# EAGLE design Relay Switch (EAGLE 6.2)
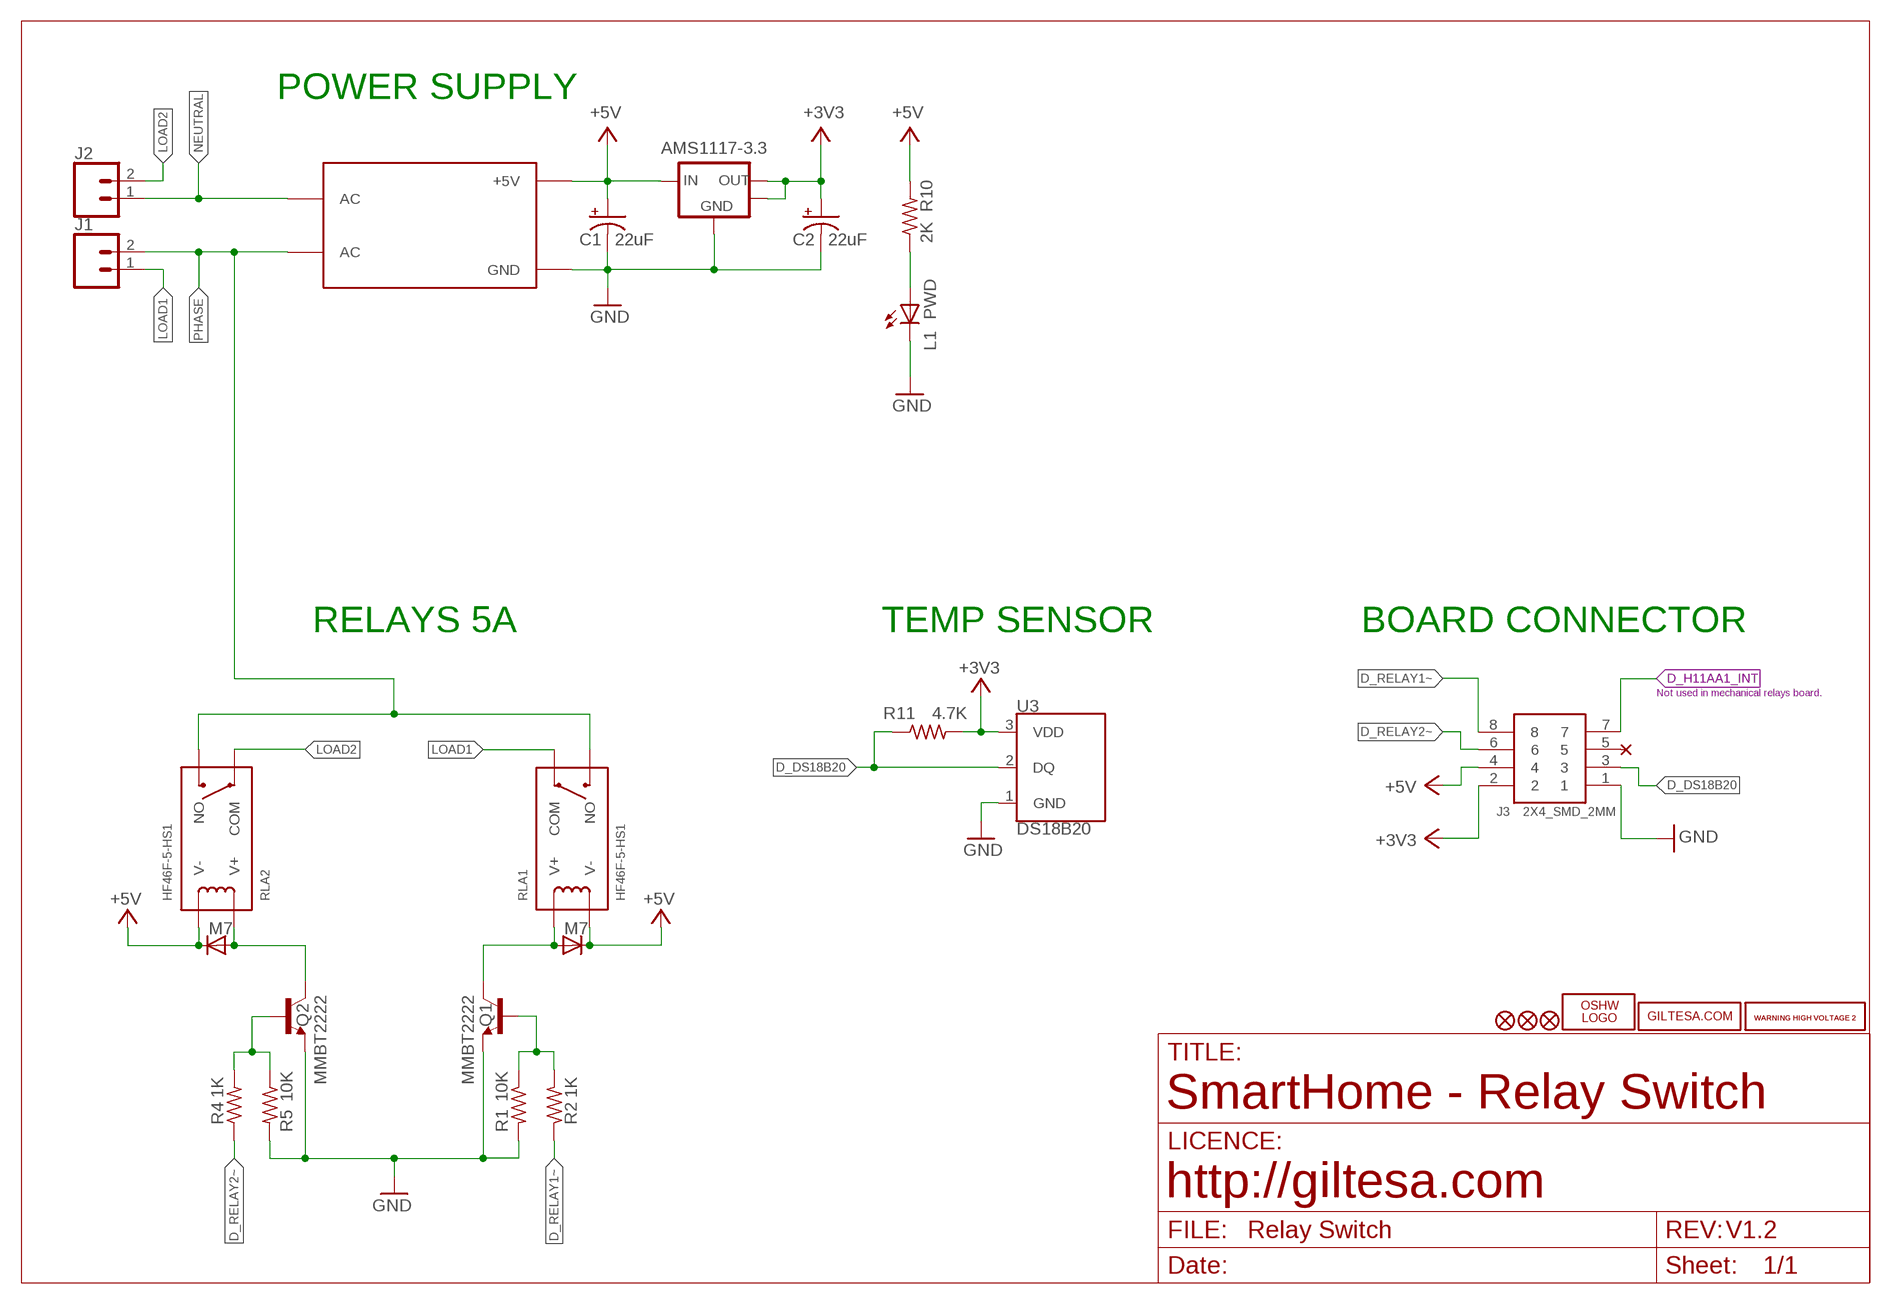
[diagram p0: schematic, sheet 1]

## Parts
AMS1117-3.3  AMS1117-3.3  AMS1117SOT89_2  [SOT89_2]
C1  22uF  CAP_POL3528  [EIA3528]
C2  22uF  CAP_POL3528  [EIA3528]
D1  M7  DIODE-SMB  [SMB]
D2  M7  DIODE-SMB  [SMB]
J1  TERMINAL_5MM_2P_90º  [TERMINAL_5MM_2P_90º]
J2  TERMINAL_5MM_2P_90º  [TERMINAL_5MM_2P_90º]
J3  2X4_SMD_2MM  2X4_SMD_2.0MM  [2X4_SMD_2.0MM]
L1  PWD  LEDCHIP-LED0805  [CHIP-LED0805]
LOGO1  OSHW_LOGO_FILLX0150-NT  [OSHW_FILLX150_NOTEXT]
Q1  MMBT2222  TRANSISTOR_NPNSOT23  [SOT23]
Q2  MMBT2222  TRANSISTOR_NPNSOT23  [SOT23]
R1  10K  R0603  [R0603]
R2  1K  R0603  [R0603]
R4  1K  R0603  [R0603]
R5  10K  R0603  [R0603]
R10  2K  R0603  [R0603]
R11  4.7K  R0603  [R0603]
RLA1  HF46F-5-HS1  RELAY_HF46F-5-HS1  [RELAY_HF46F-5-HS1]
RLA2  HF46F-5-HS1  RELAY_HF46F-5-HS1  [RELAY_HF46F-5-HS1]
U3  DS18B20  [DS18B20]
U$1  HILINK_HLK-PM01_5V  [HILINK_HLK-PM01_5V]
U$3  WARNING_HIGH_VOLTAGE_2  [WARNING_HIGH_VOLTAGE_2]
U$4  WARNING_HIGH_VOLTAGE_2  [WARNING_HIGH_VOLTAGE_2]
U$5  GILTESA.COM_MASK  [GILTESA.COM_MASK]
U$6  FIDUCIAL1X2  [FIDUCIAL-1X2]
U$7  FIDUCIAL1X2  [FIDUCIAL-1X2]
U$14  FIDUCIAL1X2  [FIDUCIAL-1X2]

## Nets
+3V3: AMS1117-3.3.2(OUT) AMS1117-3.3.4(NC) C2.A(+) J3.2 R11.2 U3.3(VDD)
+5V: AMS1117-3.3.3(IN) C1.A(+) D1.C D2.C J3.4 R10.2 RLA1.V- RLA2.V- U$1.+5V
D_DS18B20: J3.3 R11.1 U3.2(DQ)
D_H11AA1_INT: J3.7
D_RELAY1~: J3.8 R2.1
D_RELAY2~: J3.6 R4.1
GND: AMS1117-3.3.1(GND) C1.C(-) C2.C(-) J3.1 L1.C Q1.2(E) Q2.2(E) R1.2 R5.2 U3.1(GND) U$1.GND
LOAD1: J1.1 RLA1.COM
LOAD2: J2.2 RLA2.COM
N$2: Q1.1(B) R1.1 R2.2
N$3: D1.A Q1.3(C) RLA1.V+
N$8: L1.A R10.1
N$46: Q2.1(B) R4.2 R5.1
N$47: D2.A Q2.3(C) RLA2.V+
NEUTRAL: J2.1 U$1.AC@2(AC)
PHASE: J1.2 RLA1.NO RLA2.NO U$1.AC@1(AC)
Unconnected: J3.5

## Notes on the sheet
- POWER SUPPLY
- RELAYS 5A | TEMP SENSOR | BOARD CONNECTOR
- Not used in mechanical relays board.
- SmartHome - Relay Switch
- http://giltesa.com
- V1.2

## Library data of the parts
AMS1117-3.3 = ,giltesa:AMS1117
C1 C2 = SparkFun:CAP_POL: Capacitor Polarized
D1 D2 = diode:DIODE-: DIODE
J1 J2 = ,giltesa:TERMINAL_5MM_2P_90º
J3 = ,giltesa:2X4_SMD_2.0MM
L1 = led:LED: LED
LOGO1 = ohw-logo:OSHW_LOGO_FILL
Q1 Q2 = SparkFun:TRANSISTOR_NPN: Transistor NPN BJT configuration in SOT23 package. MMBT2222 is the common NPN we use. Double check BCE configuration again layout.
R1 R2 R4 R5 R10 R11 = ,giltesa:R0603
RLA1 RLA2 = ,giltesa:RELAY_HF46F-5-HS1
U3 = ,giltesa:DS18B20
U$1 = ,giltesa:HILINK_HLK-PM01_5V
U$3 U$4 = ,giltesa_logos:WARNING_HIGH_VOLTAGE_2
U$5 = ,giltesa_logos:GILTESA.COM_MASK
U$6 U$7 U$14 = SparkFun:FIDUCIAL: Fiducial Alignment Points

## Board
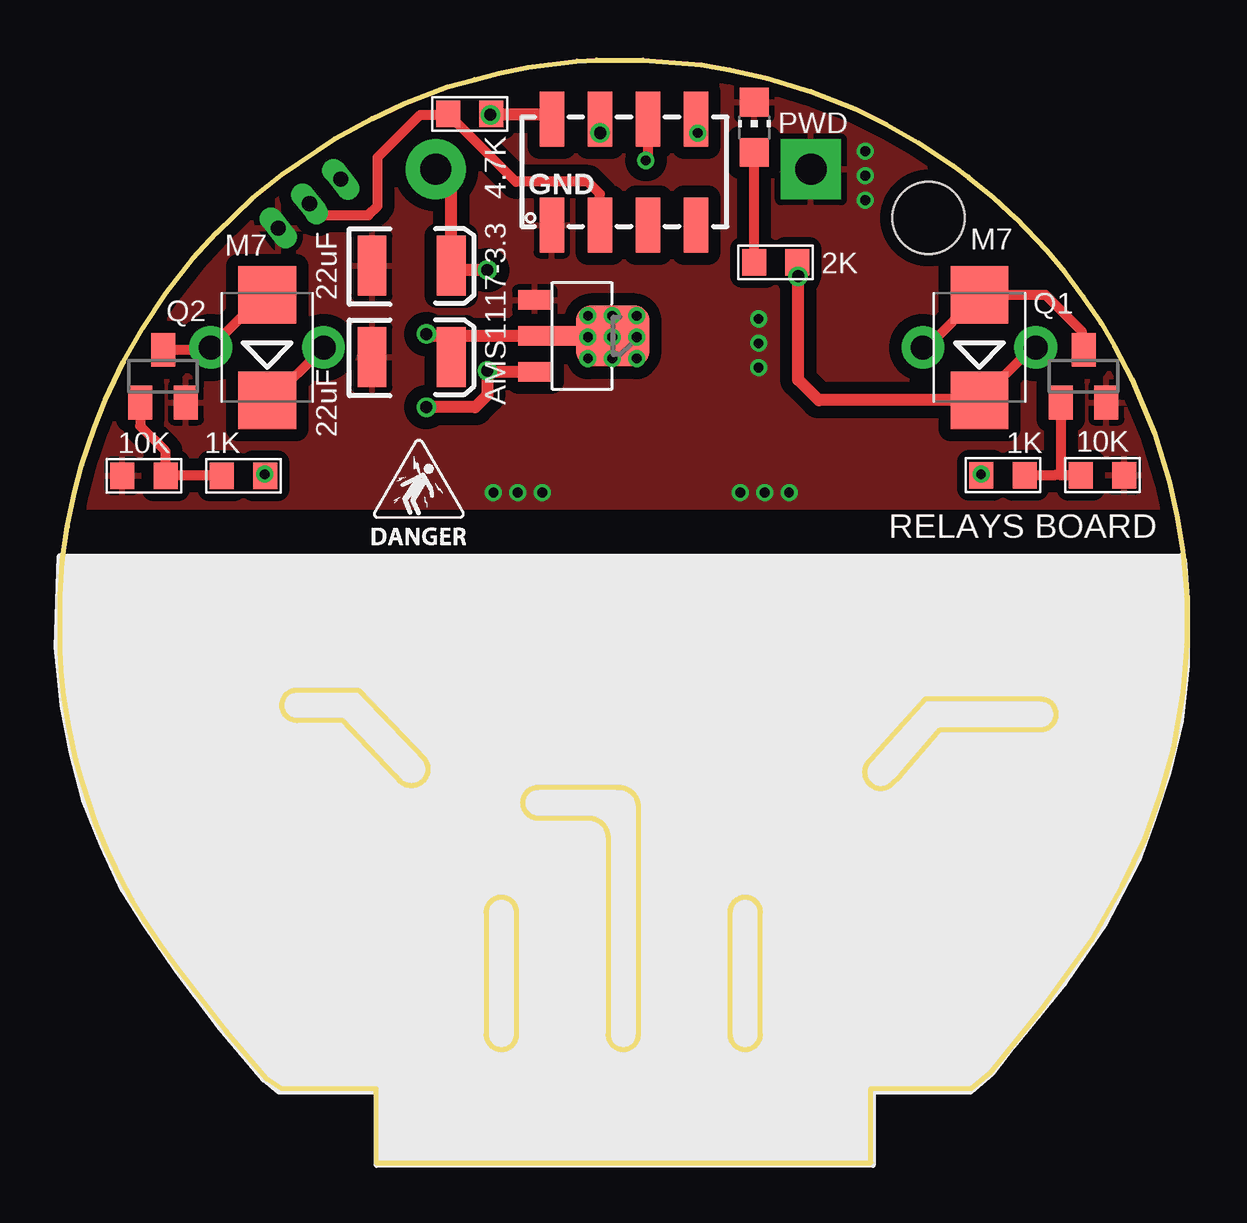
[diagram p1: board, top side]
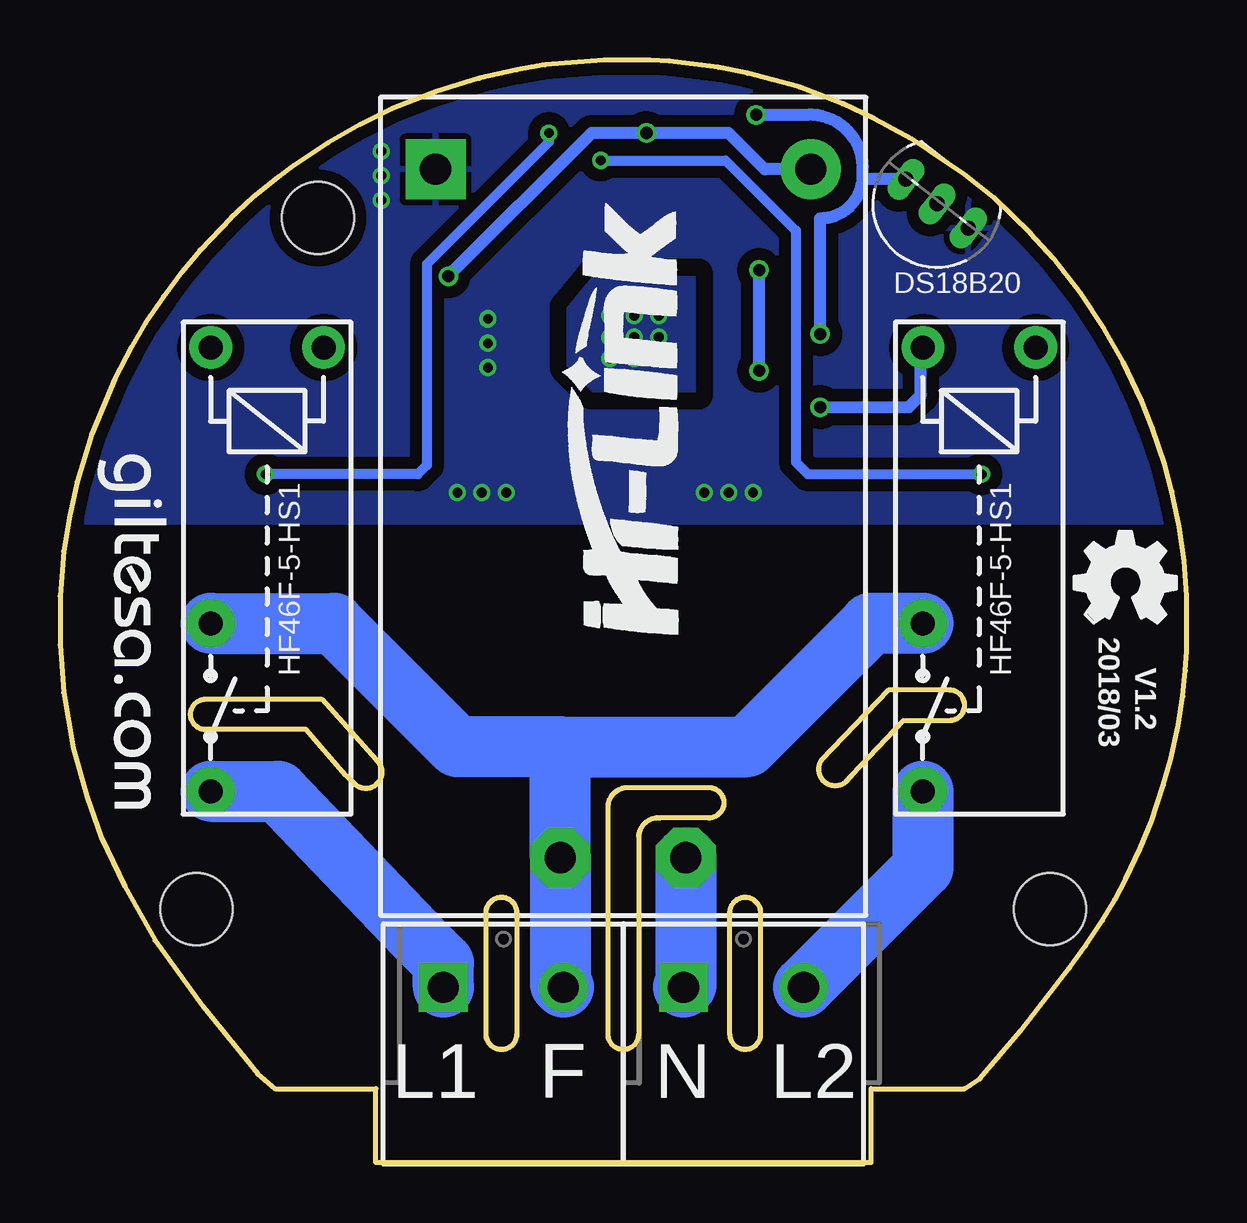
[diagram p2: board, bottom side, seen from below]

Size 46.94 x 45.97 mm. Coordinates in mm from the lower left corner, seen from the top.
Outline: 107 segments
Copper layers (1*16): Top 0.035mm / dielectric 1.6mm / Bottom 0.035mm
Design rules: minimum track width 6mil, minimum drill 12mil, track to track 6mil, track to pad 6mil, pad to pad 6mil, via to via 8mil, smd to smd 0mil, copper to edge 20mil, drill to drill 10mil, minimum pad ring 6mil, minimum via ring 6mil, stop-mask expansion 0mil, vias tented up to drill 100mil, thermal gap 10mil
Holes 3 mm at 5.69,10.57 41.25,10.57 36.19,39.38
bRestrict: 6 lines

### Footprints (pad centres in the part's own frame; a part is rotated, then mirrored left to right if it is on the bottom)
SOT89_2 = smd 0.8 x 1.4: 1 -1.499,-1.981; 3 1.499,-1.981 | smd 0.8 x 2.54: 2 0,-1.409 | smd 2.54 x 3.048: 4 0,1.27
EIA3528 = smd 1.2 x 2.5: A 1.65,0; C -1.65,0
SMB = smd 2.4 x 2.4: A 2.2,0; C -2.2,0
TERMINAL_5MM_2P_90º = drill 1.3 pad 2.032 square: 1 0.004,0 | drill 1.3 pad 2.032: 2 5.004,0
2X4_SMD_2.0MM = smd 2.286 x 1.016: 1 -2.213,2.976; 2 2.212,2.976; 3 -2.213,0.976; 4 2.212,0.976; 5 -2.213,-1.024; 6 2.212,-1.024; 7 -2.213,-3.024; 8 2.212,-3.024
CHIP-LED0805 = smd 1.2 x 1.2: A 0,-1.05; C 0,1.05
SOT23 = smd 1 x 1.4: 1 -0.95,-1.1; 2 0.95,-1.1; 3 0,1.1
R0603 = smd 1 x 1.1: 1 -0.901,0.013; 2 0.901,0.013
RELAY_HF46F-5-HS1 = drill 1 pad 2.032: COM 9.3,-2.35; NO 2.3,-2.35 | drill 1 pad 1.778: V+ -9.2,2.35; V- -9.2,-2.35
DS18B20 = drill 0.635 pad 0.864 long: 1 -1.651,0; 2 0,0; 3 1.651,0
HILINK_HLK-PM01_5V = drill 1.3 pad 2.5: +5V 31.109,2.3 | drill 1.3 pad 2.5 octagon: AC@1 2.409,12.73; AC@2 2.409,7.5 | drill 1.3 pad 2.5 square: GND 31.109,17.93
FIDUCIAL-1X2 = smd 1 x 1: 1 0,0

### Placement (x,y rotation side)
AMS1117-3.3  21.76,34.46 270 top
C1  14.65,37.38 0 top
C2  14.65,33.57 0 top
D1  38.3,33.98 90 top
D2  8.63,33.98 90 top
J1  30.97,7.31 0 bottom
J2  20.97,7.31 0 bottom
J3  23.47,41.29 90 top
L1  28.93,43.16 0 top
LOGO1  4.67,22.5 0 bottom
Q1  42.65,32.78 0 top
Q2  4.29,32.78 0 top
R1  43.44,28.65 0 top
R2  39.29,28.65 0 top
R4  7.65,28.65 180 top
R5  3.5,28.65 180 top
R10  29.82,37.51 0 top
R11  17.07,43.7 0 top
RLA1  38.3,24.78 270 bottom
RLA2  8.63,24.78 270 bottom
U3  10.4,39.98 142 bottom
U$1  13.36,10.3 90 bottom
U$2  [ELECTROCUTION_SMALL]  12.76,25.63 0 top
U$3  0.48,15.51 0 top
U$4  43.03,15.51 0 top
U$5  45.44,29.61 270 bottom
U$6  32.42,1.37 90 top
U$7  14.54,1.37 90 top
U$14  23.47,24.66 90 top

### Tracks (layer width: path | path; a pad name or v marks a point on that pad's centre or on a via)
+3V3  (via drill 0.41, 0.51)
  Top 0.406: AMS1117-3.3.2 21.95,34.46 v22,34.41 | v23.01,34.41 23.01,34.44 AMS1117-3.3.4
  Top 0.508: AMS1117-3.3.2 16.41,34.46 | 16.41,34.46 15.34,34.46 v15.27,34.54 | C2.A 16.3,34.36 16.41,34.46 | J3.2 20.49,43.66 20.47,43.68 v17.93,43.68 18.03,43.71 R11.2
  Bottom 0.508: v15.27,34.54 15.27,39.37 arc-90 13.49,41.14 | v17.93,43.68 15.77,43.68 arc90 13.49,41.52 13.49,41.14 | U3.3 13.34,40.99 arc90 13.49,41.14
  other vias: 22,35.3 23.01,35.3 24.03,35.3 24.03,34.41 24.03,33.52 23.01,33.52 22,33.52
  pour Bottom: 20.47,32 20.47,36.95 24.79,36.95 25.81,35.68 25.81,33.14 24.79,32
+5V  (via drill 0.51)
  Top 0.406: D1.C 40.51,33.98 RLA1.V- | D2.C 8.78,31.78 RLA2.V-
  Top 0.508: U$1.+5V 16.3,40.77 C1.A 16.48,37.21 v17.81,37.21 | R10.2 30.76,37.49 v30.76,36.95 30.76,32.63 31.61,31.78 D1.C | J3.4 22.49,42.91 v22.5,42.92 | v15.27,31.49 17.3,31.49 17.81,32 v17.81,33.02 17.88,32.96 AMS1117-3.3.3
  Bottom 0.508: v17.81,33.02 v17.81,37.21 | U$1.+5V 17.57,41.41 19.08,42.92 v22.5,42.92 24.79,42.92 v30.76,36.95 | v15.27,31.49 11.58,31.49 11.07,32 11.07,33.89 RLA2.V-
D_DS18B20
  Top 0.406: U3.2 10.46,39.98 10.95,39.49 12.85,39.49 13.23,39.87 13.23,41.91 15.01,43.68 16.14,43.68 R11.1 19,40.89 22,40.89 22.49,40.39 J3.3
D_RELAY1~  (via drill 0.41)
  Top 0.406: J3.8 26.49,42.97 26.44,42.92 v26.57,42.92 | v38.38,28.7 38.3,28.57 R2.1
  Bottom 0.406: v26.57,42.92 26.57,42.54 31.65,37.46 31.65,29.08 32.03,28.7 v38.38,28.7
D_RELAY2~  (via drill 0.41)
  Top 0.406: J3.6 24.49,41.86 v24.41,41.78 | v8.53,28.7 8.61,28.7 R4.1
  Bottom 0.406: v24.41,41.78 19.2,41.78 16.28,38.86 16.28,29.21 15.77,28.7 v8.53,28.7
GND  (via drill 0.41)
  other vias: 29.11,35.17 29.11,34.16 29.11,33.14 18.06,27.94 19.08,27.94 20.09,27.94 30.38,27.94 29.36,27.94 28.35,27.94 33.55,42.16 33.55,41.14 33.55,40.13
  pour Top (isolate 0.508): -0.03,27.32 46.96,27.32 46.96,27.58 46.33,28.85 45.06,32.02 42.52,36.47 39.98,39.64 35.53,42.82 29.82,45.36 24.74,45.99 20.93,45.99 15.85,44.72 10.77,42.18 6.96,39.01 3.78,35.2 1.88,32.02 0.61,28.21
  pour Bottom (isolate 0.508): -0.03,26.69 46.96,26.69 46.33,28.85 45.06,32.02 42.52,36.47 39.98,39.64 35.53,42.82 29.82,45.36 24.74,45.99 20.93,45.99 15.85,44.72 10.77,42.18 6.96,39.01 3.78,35.2 1.88,32.02
LOAD1
  Bottom 2.54: RLA1.COM 37.86,15.48 32.16,9.52 30.97,8.33 J1.1
LOAD2
  Bottom 2.54: RLA2.COM 10.98,12.29 J2.2
N$2
  Top 0.406: R2.2 41.43,28.66 41.7,28.66 | 41.7,28.66 R1.1 | Q1.1 41.7,28.66
N$3
  Top 0.406: RLA1.V+ 36.11,33.98 D1.A 41.06,36.18 42.57,34.67 42.57,33.96 Q1.3
N$8
  Top 0.406: R10.1 28.92,42.1 L1.A
N$46
  Top 0.406: R4.2 R5.1 4.4,29.65 3.34,30.71 Q2.1
N$47
  Top 0.406: Q2.3 6.19,33.88 RLA2.V+ 8.48,36.18 D2.A
NEUTRAL
  Bottom 2.54: U$1.AC@2 20.86,7.41 J2.1
PHASE
  Bottom 2.54: 26.09,17.34 U$1.AC@1 26.09,7.44 J1.2 | 26.09,17.34 18.31,17.34 13.17,22.48 RLA2.NO | 26.09,17.34 30.38,17.34 35.53,22.48 RLA1.NO

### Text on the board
tPlace: GND | RELAYS BOARD
bPlace: 2018/03 | V1.2 | L2 | N | F | L1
